DATA_BLOCK "DB_STATUS_OP37"
TITLE =BLOCK DATA FOR STATUS MONITOR PAGE PRESS OP_37
AUTHOR : Esposito
FAMILY : EGAL_srl
NAME : DB_STATU
VERSION : 0.1


  STRUCT
   Menu_press0 : BOOL ;	//Spare munu press monitor for OP_37
   Menu_press1 : BOOL ;	//Spare munu press monitor for OP_37
   Menu_press2 : BOOL ;	//Spare munu press monitor for OP_37
   Menu_press3 : BOOL ;	//Spare munu press monitor for OP_37
   Menu_press4 : BOOL ;	//Spare munu press monitor for OP_37
   Menu_press5 : BOOL ;	//Spare munu press monitor for OP_37
   Menu_press6 : BOOL ;	//Spare munu press monitor for OP_37
   Menu_press7 : BOOL ;	//Spare munu press monitor for OP_37
   Menu_press8 : BOOL ;	//Spare munu press monitor for OP_37
   Menu_press9 : BOOL ;	//Spare munu press monitor for OP_37
   Menu_press10 : BOOL ;	//Spare munu press monitor for OP_37
   Menu_press11 : BOOL ;	//Spare munu press monitor for OP_37
   Menu_press12 : BOOL ;	//Spare munu press monitor for OP_37
   Menu_press13 : BOOL ;	//Spare munu press monitor for OP_37
   Menu_press14 : BOOL ;	//Spare munu press monitor for OP_37
   Menu_press15 : BOOL ;	//Spare munu press monitor for OP_37
   Menu_line0 : BOOL ;	//Spare menu line monitor for OP_37
   Menu_line1 : BOOL ;	//Spare menu line monitor for OP_37
   Menu_line2 : BOOL ;	//Spare menu line monitor for OP_37
   Menu_line3 : BOOL ;	//Spare menu line monitor for OP_37
   Menu_line4 : BOOL ;	//Spare menu line monitor for OP_37
   Menu_line5 : BOOL ;	//Spare menu line monitor for OP_37
   Menu_line6 : BOOL ;	//Spare menu line monitor for OP_37
   Menu_line7 : BOOL ;	//Spare menu line monitor for OP_37
   Menu_line8 : BOOL ;	//Spare menu line monitor for OP_37
   Menu_line9 : BOOL ;	//Spare menu line monitor for OP_37
   Menu_line10 : BOOL ;	//Spare menu line monitor for OP_37
   Menu_line11 : BOOL ;	//Spare menu line monitor for OP_37
   Menu_line12 : BOOL ;	//Spare menu line monitor for OP_37
   Menu_line13 : BOOL ;	//Spare menu line monitor for OP_37
   Menu_line14 : BOOL ;	//Spare menu line monitor for OP_37
   Menu_line15 : BOOL ;	//Spare menu line monitor for OP_37
   Menu_setup0 : BOOL ;
   Menu_setup1 : BOOL ;
   Menu_setup2 : BOOL ;
   Menu_setup3 : BOOL ;
   Menu_setup4 : BOOL ;
   Menu_setup5 : BOOL ;
   Menu_setup6 : BOOL ;
   Menu_setup7 : BOOL ;
   Menu_setup8 : BOOL ;
   Menu_setup9 : BOOL ;
   Menu_setup10 : BOOL ;
   Menu_setup11 : BOOL ;
   Menu_setup12 : BOOL ;
   Menu_setup13 : BOOL ;
   Menu_setup14 : BOOL ;
   Menu_setup15 : BOOL ;
   Main_press0 : BOOL ;
   Main_press1 : BOOL ;
   Main_press2 : BOOL ;
   Main_press3 : BOOL ;
   Main_press4 : BOOL ;
   Main_press5 : BOOL ;
   Main_press6 : BOOL ;
   Main_press7 : BOOL ;
   Main_press8 : BOOL ;
   Main_press9 : BOOL ;
   Main_press10 : BOOL ;
   Main_press11 : BOOL ;
   Main_press12 : BOOL ;
   Main_press13 : BOOL ;
   Main_press14 : BOOL ;
   Main_press15 : BOOL ;
   Motor_pr0 : BOOL ;
   Motor_pr1 : BOOL ;
   Motor_pr2 : BOOL ;
   Motor_pr3 : BOOL ;
   Motor_pr4 : BOOL ;
   Motor_pr5 : BOOL ;
   Motor_pr6 : BOOL ;
   Motor_pr7 : BOOL ;
   Motor_pr8 : BOOL ;
   Motor_pr9 : BOOL ;
   Motor_pr10 : BOOL ;
   Motor_pr11 : BOOL ;
   Motor_pr12 : BOOL ;
   Motor_pr13 : BOOL ;
   Motor_pr14 : BOOL ;
   Motor_pr15 : BOOL ;
   Slide_adj0 : BOOL ;	//Auxiliaris ON press
   Slide_adj1 : BOOL ;	//Emergencies OFF
   Slide_adj2 : BOOL ;	//Press in Inching mode ON
   Slide_adj3 : BOOL ;	//Selector switch - enable adjustment mode
   Slide_adj4 : BOOL ;	//Circuit clutch/brake OFF
   Slide_adj5 : BOOL ;	//Safety jack OFF
   Slide_adj6 : BOOL ;	//Spare slide adjustment monitor for OP_37
   Slide_adj7 : BOOL ;	//Spare slide adjustment monitor for OP_37
   Slide_adj8 : BOOL ;	//Alarm slide adjustment
   Slide_adj9 : BOOL ;	//Wagon in position
   Slide_adj10 : BOOL ;	//Press in UDP
   Slide_adj11 : BOOL ;	//Upper limit switch slide adjustment
   Slide_adj12 : BOOL ;	//Lower limit switch slide sdjustment
   Slide_adj13 : BOOL ;	//Spare slide adjustment monitor for OP_37
   Slide_adj14 : BOOL ;	//Spare slide adjustment monitor for OP_37
   Slide_adj15 : BOOL ;	//Spare slide adjustment monitor for OP_37
   Lubrication_0 : BOOL ;	//Pomp lubrication oil in Run
   Lubrication_1 : BOOL ;	//Pomp Torc_Pac in Run
   Lubrication_2 : BOOL ;	//Pomp balance in Run
   Lubrication_3 : BOOL ;	//Pomp balance in Automatic
   Lubrication_4 : BOOL ;	//Pomp balance in Manual
   Lubrication_5 : BOOL ;	//Spare lubrication monitor for OP_37
   Lubrication_6 : BOOL ;	//Spare lubrication monitor for OP_37
   Lubrication_7 : BOOL ;	//Spare lubrication monitor for OP_37
   Lubrication_8 : BOOL ;	//Alarm pomp lubrication oil
   Lubrication_9 : BOOL ;	//Alarm pomp Torc_pac press
   Lubrication_10 : BOOL ;	//Alarm pomp lubrication balancing
   Lubrication_11 : BOOL ;	//Spare lubrication monitor for OP_37
   Lubrication_12 : BOOL ;	//Spare lubrication monitor for OP_37
   Lubrication_13 : BOOL ;	//Spare lubrication monitor for OP_37
   Lubrication_14 : BOOL ;	//Spare lubrication monitor for OP_37
   Lubrication_15 : BOOL ;	//Spare lubrication monitor for OP_37
   Overload_0 : BOOL ;	//Maximal pressure overload
   Overload_1 : BOOL ;	//Minimal pressure overload
   Overload_2 : BOOL ;	//Electrical valve air pomp overload ON
   Overload_3 : BOOL ;	//Electrical valve oil safety overload ON
   Overload_4 : BOOL ;	//Spare overload monitor for OP_37
   Overload_5 : BOOL ;	//Spare overload monitor for OP_37
   Overload_6 : BOOL ;	//Spare overload monitor for OP_37
   Overload_7 : BOOL ;	//Spare overload monitor for OP_37
   Overload_8 : BOOL ;	//Not alarm overload
   Overload_9 : BOOL ;	//Alarm proportional valve
   Overload_10 : BOOL ;	//Spare overload monitor for OP_37
   Overload_11 : BOOL ;	//Spare overload monitor for OP_37
   Overload_12 : BOOL ;	//Spare overload monitor for OP_37
   Overload_13 : BOOL ;	//Spare overload monitor for OP_37
   Overload_14 : BOOL ;	//Spare overload monitor for OP_37
   Overload_15 : BOOL ;	//Spare overload monitor for OP_37
   Balances_0 : BOOL ;	//Maximal tonnage balances
   Balances_1 : BOOL ;	//Minimal tonnage balances
   Balances_2 : BOOL ;	//Minimal pressure balances
   Balances_3 : BOOL ;	//Not alarm balances
   Balances_4 : BOOL ;	//Spare balances monitor for OP_37
   Balances_5 : BOOL ;	//Spare balances monitor for OP_37
   Balances_6 : BOOL ;	//Spare balances monitor for OP_37
   Balances_7 : BOOL ;	//Spare balances monitor for OP_37
   Balances_8 : BOOL ;	//Electrical valve load balances ON
   Balances_9 : BOOL ;	//Electrical valve unload balances ON
   Balances_10 : BOOL ;	//Spare balances monitor for OP_37
   Balances_11 : BOOL ;	//Spare balances monitor for OP_37
   Balances_12 : BOOL ;	//Spare balances monitor for OP_37
   Balances_13 : BOOL ;	//Spare balances monitor for OP_37
   Balances_14 : BOOL ;	//Spare balances monitor for OP_37
   Balances_15 : BOOL ;	//Spare balances monitor for OP_37
   Cams_elec0 : BOOL ;
   Cams_elec1 : BOOL ;
   Cams_elec2 : BOOL ;
   Cams_elec3 : BOOL ;
   Cams_elec4 : BOOL ;
   Cams_elec5 : BOOL ;
   Cams_elec6 : BOOL ;
   Cams_elec7 : BOOL ;
   Cams_elec8 : BOOL ;
   Cams_elec9 : BOOL ;
   Cams_elec10 : BOOL ;
   Cams_elec11 : BOOL ;
   Cams_elec12 : BOOL ;
   Cams_elec13 : BOOL ;
   Cams_elec14 : BOOL ;
   Cams_elec15 : BOOL ;
   Cams_plc0 : BOOL ;
   Cams_plc1 : BOOL ;
   Cams_plc2 : BOOL ;
   Cams_plc3 : BOOL ;
   Cams_plc4 : BOOL ;
   Cams_plc5 : BOOL ;
   Cams_plc6 : BOOL ;
   Cams_plc7 : BOOL ;
   Cams_plc8 : BOOL ;
   Cams_plc9 : BOOL ;
   Cams_plc10 : BOOL ;
   Cams_plc11 : BOOL ;
   Cams_plc12 : BOOL ;
   Cams_plc13 : BOOL ;
   Cams_plc14 : BOOL ;
   Cams_plc15 : BOOL ;
   Counter_0 : BOOL ;
   Counter_1 : BOOL ;
   Counter_2 : BOOL ;
   Counter_3 : BOOL ;
   Counter_4 : BOOL ;
   Counter_5 : BOOL ;
   Counter_6 : BOOL ;
   Counter_7 : BOOL ;
   Counter_8 : BOOL ;
   Counter_9 : BOOL ;
   Counter_10 : BOOL ;
   Counter_11 : BOOL ;
   Counter_12 : BOOL ;
   Counter_13 : BOOL ;
   Counter_14 : BOOL ;
   Counter_15 : BOOL ;
   Inlets_0 : BOOL ;	//Running inlet one from PLC press
   Inlets_1 : BOOL ;	//Running inlet two from PLC press
   Inlets_2 : BOOL ;	//Running inlet three from PLC press
   Inlets_3 : BOOL ;	//Running inlet four from PLC press
   Inlets_4 : BOOL ;	//Spare Inlets monitor for OP_37
   Inlets_5 : BOOL ;	//Spare Inlets monitor for OP_37
   Inlets_6 : BOOL ;	//Spare Inlets monitor for OP_37
   Inlets_7 : BOOL ;	//Spare Inlets monitor for OP_37
   Inlets_8 : BOOL ;	//Not alarm inlet one from PLC press
   Inlets_9 : BOOL ;	//Not alarm inlet two from PLC press
   Inlets_10 : BOOL ;	//Not alarm inlet three from PLC press
   Inlets_11 : BOOL ;	//Not alarm inlet four from PLC press
   Inlets_12 : BOOL ;	//Spare Inlets monitor for OP_37
   Inlets_13 : BOOL ;	//Spare Inlets monitor for OP_37
   Inlets_14 : BOOL ;	//Spare Inlets monitor for OP_37
   Inlets_15 : BOOL ;	//Spare Inlets monitor for OP_37
   Die_change0 : BOOL ;
   Die_change1 : BOOL ;
   Die_change2 : BOOL ;
   Die_change3 : BOOL ;
   Die_change4 : BOOL ;
   Die_change5 : BOOL ;
   Die_change6 : BOOL ;
   Die_change7 : BOOL ;
   Die_change8 : BOOL ;
   Die_change9 : BOOL ;
   Die_change10 : BOOL ;
   Die_change11 : BOOL ;
   Die_change12 : BOOL ;
   Die_change13 : BOOL ;
   Die_change14 : BOOL ;
   Die_change15 : BOOL ;
   Die_safety0 : BOOL ;
   Die_safety1 : BOOL ;
   Die_safety2 : BOOL ;
   Die_safety3 : BOOL ;
   Die_safety4 : BOOL ;
   Die_safety5 : BOOL ;
   Die_safety6 : BOOL ;
   Die_safety7 : BOOL ;
   Die_safety8 : BOOL ;
   Die_safety9 : BOOL ;
   Die_safety10 : BOOL ;
   Die_safety11 : BOOL ;
   Die_safety12 : BOOL ;
   Die_safety13 : BOOL ;
   Die_safety14 : BOOL ;
   Die_safety15 : BOOL ;
   Robot1_robot2 : BOOL ;	//Segnale robot 1 - robot 2
   Pallet1_pallet2 : BOOL ;	//Segnale pallet 1- pallet 2
   Pallet2_pallet1 : BOOL ;	//Segnale pallet 2- pallet 1
   Robot_1 : BOOL ;	//Segnale robot 1
   Robot_2 : BOOL ;	//Segnale robot 2
   FEEDER_TAVOLA : BOOL ;	//Segnale comando feeder da tavola
   FEEDER_PRESSA : BOOL ;	//Segnale comando feeder da pressa
   Spare_OP7 : BOOL ;
   Spare_OP8 : BOOL ;
   Spare_OP9 : BOOL ;
   Spare_OP10 : BOOL ;
   Spare_OP11 : BOOL ;
   Spare_OP12 : BOOL ;
   Spare_OP13 : BOOL ;
   Spare_OP14 : BOOL ;
   Spare_OP15 : BOOL ;
  END_STRUCT ;
BEGIN
   Menu_press0 := FALSE;
   Menu_press1 := FALSE;
   Menu_press2 := FALSE;
   Menu_press3 := FALSE;
   Menu_press4 := FALSE;
   Menu_press5 := FALSE;
   Menu_press6 := FALSE;
   Menu_press7 := FALSE;
   Menu_press8 := FALSE;
   Menu_press9 := FALSE;
   Menu_press10 := FALSE;
   Menu_press11 := FALSE;
   Menu_press12 := FALSE;
   Menu_press13 := FALSE;
   Menu_press14 := FALSE;
   Menu_press15 := FALSE;
   Menu_line0 := FALSE;
   Menu_line1 := FALSE;
   Menu_line2 := FALSE;
   Menu_line3 := FALSE;
   Menu_line4 := FALSE;
   Menu_line5 := FALSE;
   Menu_line6 := FALSE;
   Menu_line7 := FALSE;
   Menu_line8 := FALSE;
   Menu_line9 := FALSE;
   Menu_line10 := FALSE;
   Menu_line11 := FALSE;
   Menu_line12 := FALSE;
   Menu_line13 := FALSE;
   Menu_line14 := FALSE;
   Menu_line15 := FALSE;
   Menu_setup0 := FALSE;
   Menu_setup1 := FALSE;
   Menu_setup2 := FALSE;
   Menu_setup3 := FALSE;
   Menu_setup4 := FALSE;
   Menu_setup5 := FALSE;
   Menu_setup6 := FALSE;
   Menu_setup7 := FALSE;
   Menu_setup8 := FALSE;
   Menu_setup9 := FALSE;
   Menu_setup10 := FALSE;
   Menu_setup11 := FALSE;
   Menu_setup12 := FALSE;
   Menu_setup13 := FALSE;
   Menu_setup14 := FALSE;
   Menu_setup15 := FALSE;
   Main_press0 := FALSE;
   Main_press1 := FALSE;
   Main_press2 := FALSE;
   Main_press3 := FALSE;
   Main_press4 := FALSE;
   Main_press5 := FALSE;
   Main_press6 := FALSE;
   Main_press7 := FALSE;
   Main_press8 := FALSE;
   Main_press9 := FALSE;
   Main_press10 := FALSE;
   Main_press11 := FALSE;
   Main_press12 := FALSE;
   Main_press13 := FALSE;
   Main_press14 := FALSE;
   Main_press15 := FALSE;
   Motor_pr0 := FALSE;
   Motor_pr1 := FALSE;
   Motor_pr2 := FALSE;
   Motor_pr3 := FALSE;
   Motor_pr4 := FALSE;
   Motor_pr5 := FALSE;
   Motor_pr6 := FALSE;
   Motor_pr7 := FALSE;
   Motor_pr8 := FALSE;
   Motor_pr9 := FALSE;
   Motor_pr10 := FALSE;
   Motor_pr11 := FALSE;
   Motor_pr12 := FALSE;
   Motor_pr13 := FALSE;
   Motor_pr14 := FALSE;
   Motor_pr15 := FALSE;
   Slide_adj0 := FALSE;
   Slide_adj1 := FALSE;
   Slide_adj2 := FALSE;
   Slide_adj3 := FALSE;
   Slide_adj4 := FALSE;
   Slide_adj5 := FALSE;
   Slide_adj6 := FALSE;
   Slide_adj7 := FALSE;
   Slide_adj8 := FALSE;
   Slide_adj9 := FALSE;
   Slide_adj10 := FALSE;
   Slide_adj11 := FALSE;
   Slide_adj12 := FALSE;
   Slide_adj13 := FALSE;
   Slide_adj14 := FALSE;
   Slide_adj15 := FALSE;
   Lubrication_0 := FALSE;
   Lubrication_1 := FALSE;
   Lubrication_2 := FALSE;
   Lubrication_3 := FALSE;
   Lubrication_4 := FALSE;
   Lubrication_5 := FALSE;
   Lubrication_6 := FALSE;
   Lubrication_7 := FALSE;
   Lubrication_8 := FALSE;
   Lubrication_9 := FALSE;
   Lubrication_10 := FALSE;
   Lubrication_11 := FALSE;
   Lubrication_12 := FALSE;
   Lubrication_13 := FALSE;
   Lubrication_14 := FALSE;
   Lubrication_15 := FALSE;
   Overload_0 := FALSE;
   Overload_1 := FALSE;
   Overload_2 := FALSE;
   Overload_3 := FALSE;
   Overload_4 := FALSE;
   Overload_5 := FALSE;
   Overload_6 := FALSE;
   Overload_7 := FALSE;
   Overload_8 := FALSE;
   Overload_9 := FALSE;
   Overload_10 := FALSE;
   Overload_11 := FALSE;
   Overload_12 := FALSE;
   Overload_13 := FALSE;
   Overload_14 := FALSE;
   Overload_15 := FALSE;
   Balances_0 := FALSE;
   Balances_1 := FALSE;
   Balances_2 := FALSE;
   Balances_3 := FALSE;
   Balances_4 := FALSE;
   Balances_5 := FALSE;
   Balances_6 := FALSE;
   Balances_7 := FALSE;
   Balances_8 := FALSE;
   Balances_9 := FALSE;
   Balances_10 := FALSE;
   Balances_11 := FALSE;
   Balances_12 := FALSE;
   Balances_13 := FALSE;
   Balances_14 := FALSE;
   Balances_15 := FALSE;
   Cams_elec0 := FALSE;
   Cams_elec1 := FALSE;
   Cams_elec2 := FALSE;
   Cams_elec3 := FALSE;
   Cams_elec4 := FALSE;
   Cams_elec5 := FALSE;
   Cams_elec6 := FALSE;
   Cams_elec7 := FALSE;
   Cams_elec8 := FALSE;
   Cams_elec9 := FALSE;
   Cams_elec10 := FALSE;
   Cams_elec11 := FALSE;
   Cams_elec12 := FALSE;
   Cams_elec13 := FALSE;
   Cams_elec14 := FALSE;
   Cams_elec15 := FALSE;
   Cams_plc0 := FALSE;
   Cams_plc1 := FALSE;
   Cams_plc2 := FALSE;
   Cams_plc3 := FALSE;
   Cams_plc4 := FALSE;
   Cams_plc5 := FALSE;
   Cams_plc6 := FALSE;
   Cams_plc7 := FALSE;
   Cams_plc8 := FALSE;
   Cams_plc9 := FALSE;
   Cams_plc10 := FALSE;
   Cams_plc11 := FALSE;
   Cams_plc12 := FALSE;
   Cams_plc13 := FALSE;
   Cams_plc14 := FALSE;
   Cams_plc15 := FALSE;
   Counter_0 := FALSE;
   Counter_1 := FALSE;
   Counter_2 := FALSE;
   Counter_3 := FALSE;
   Counter_4 := FALSE;
   Counter_5 := FALSE;
   Counter_6 := FALSE;
   Counter_7 := FALSE;
   Counter_8 := FALSE;
   Counter_9 := FALSE;
   Counter_10 := FALSE;
   Counter_11 := FALSE;
   Counter_12 := FALSE;
   Counter_13 := FALSE;
   Counter_14 := FALSE;
   Counter_15 := FALSE;
   Inlets_0 := FALSE;
   Inlets_1 := FALSE;
   Inlets_2 := FALSE;
   Inlets_3 := FALSE;
   Inlets_4 := FALSE;
   Inlets_5 := FALSE;
   Inlets_6 := FALSE;
   Inlets_7 := FALSE;
   Inlets_8 := FALSE;
   Inlets_9 := FALSE;
   Inlets_10 := FALSE;
   Inlets_11 := FALSE;
   Inlets_12 := FALSE;
   Inlets_13 := FALSE;
   Inlets_14 := FALSE;
   Inlets_15 := FALSE;
   Die_change0 := FALSE;
   Die_change1 := FALSE;
   Die_change2 := FALSE;
   Die_change3 := FALSE;
   Die_change4 := FALSE;
   Die_change5 := FALSE;
   Die_change6 := FALSE;
   Die_change7 := FALSE;
   Die_change8 := FALSE;
   Die_change9 := FALSE;
   Die_change10 := FALSE;
   Die_change11 := FALSE;
   Die_change12 := FALSE;
   Die_change13 := FALSE;
   Die_change14 := FALSE;
   Die_change15 := FALSE;
   Die_safety0 := FALSE;
   Die_safety1 := FALSE;
   Die_safety2 := FALSE;
   Die_safety3 := FALSE;
   Die_safety4 := FALSE;
   Die_safety5 := FALSE;
   Die_safety6 := FALSE;
   Die_safety7 := FALSE;
   Die_safety8 := FALSE;
   Die_safety9 := FALSE;
   Die_safety10 := FALSE;
   Die_safety11 := FALSE;
   Die_safety12 := FALSE;
   Die_safety13 := FALSE;
   Die_safety14 := FALSE;
   Die_safety15 := FALSE;
   Robot1_robot2 := FALSE;
   Pallet1_pallet2 := FALSE;
   Pallet2_pallet1 := FALSE;
   Robot_1 := FALSE;
   Robot_2 := FALSE;
   FEEDER_TAVOLA := FALSE;
   FEEDER_PRESSA := FALSE;
   Spare_OP7 := FALSE;
   Spare_OP8 := FALSE;
   Spare_OP9 := FALSE;
   Spare_OP10 := FALSE;
   Spare_OP11 := FALSE;
   Spare_OP12 := FALSE;
   Spare_OP13 := FALSE;
   Spare_OP14 := FALSE;
   Spare_OP15 := FALSE;
END_DATA_BLOCK

